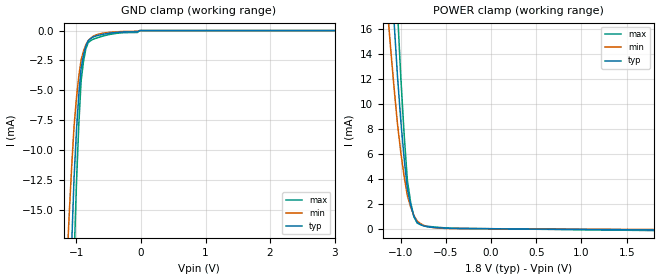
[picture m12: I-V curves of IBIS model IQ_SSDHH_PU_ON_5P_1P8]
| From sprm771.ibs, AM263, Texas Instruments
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|   Model Cell IQ_SSDHH_PU_ON_5P_1P8
|IQ_SSDHH_PU_ON_5P_1P8
[Model]   IQ_SSDHH_PU_ON_5P_1P8
Model_type   Input
Polarity   Non-Inverting
Vinl =  0.63
Vinh =  1.17
C_comp   1.313442p   1.241204p   1.780255p
|[Input load] weak_pu_on
|[supplytol] 5
|[temp] ind
[Model Spec]
Vinl   0.63   0.5985   0.6615
Vinh   1.17   1.1115   1.2285
[Temperature Range]   25   125   -40
[Voltage Range]   1.8   1.71   1.89
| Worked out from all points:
|   GND clamp passes 1 mA (typ) near -0.83 V on its own axis
|   POWER clamp passes 1 mA (typ) near -0.85 V on its own axis
| Nom Voltages:
|   VDD=1.1, VDDS=1.8, VDDS18=1.8, BUS_VSSS=0, ESD_BIASFET=0, VSS=0
| Min Voltages:
|   VDD=1.045, VDDS=1.71, VDDS18=1.71, BUS_VSSS=0, ESD_BIASFET=0, VSS=0
| Max Voltages:
|   VDD=1.16, VDDS=1.89, VDDS18=1.89, BUS_VSSS=0, ESD_BIASFET=0, VSS=0
[POWER_clamp]
|   voltage   I(typ)   I(min)   I(max)
-1.8V     125.7mA    90.96mA    174.2mA
-1.145V   25.64mA    17.42mA    36.91mA
-1.109V   20.95mA    14.21mA    30.19mA
-1.073V   16.48mA    11.21mA    23.73mA
-1.036V   12.25mA    8.409mA    17.54mA
-1V       8.723mA    6.157mA    12.23mA
-963.6mV  5.718mA    4.242mA    7.69mA
-927.3mV  3.233mA    2.665mA    3.916mA
-890.9mV  1.918mA    1.747mA    2.121mA
-818.2mV  499.9uA    614uA      454.7uA
-527.3mV  56.53uA    34.13uA    79.16uA
1.8V      -99.93uA   -59.09uA   -145.1uA
[GND_clamp]
|   voltage   I(typ)   I(min)   I(max)
-1.8V     -190.2mA   -126mA     -287.6mA
-1.145V   -30.74mA   -19.28mA   -48.29mA
-1.109V   -23.94mA   -15.08mA   -37.56mA
-1.073V   -17.79mA   -11.31mA   -27.83mA
-1.036V   -12.29mA   -7.981mA   -19.08mA
-1V       -8.448mA   -5.671mA   -12.88mA
-963.6mV  -5.397mA   -3.83mA    -7.919mA
-927.3mV  -3.136mA   -2.456mA   -4.192mA
-854.5mV  -1.305mA   -1.199mA   -1.535mA
-745.5mV  -545.3uA   -499uA     -737uA
-18.18mV  0A         0A         0A
3.6V      0A         0A         0A
